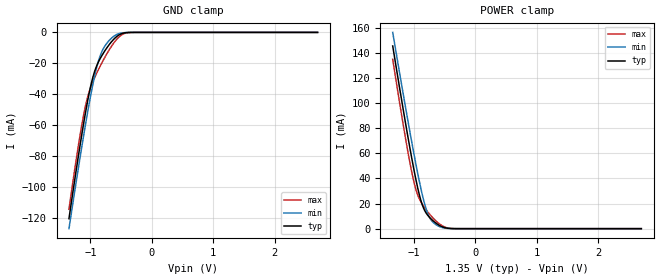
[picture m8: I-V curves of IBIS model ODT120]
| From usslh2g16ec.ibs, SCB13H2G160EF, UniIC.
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|   Model ODT120
[Model]  ODT120
Model_type Input
Vinl =   0.5750V
Vinh =   0.7750V
| variable   typ   min   max
C_comp   1.0500pF   1.0000pF   1.1000pF
| variable   typ   min   max
[Temperature Range]   45.000   95.000   0.000
| variable   typ   min   max
[Voltage Range]   1.35V   1.283V   1.4250V
| variable   typ   min   max
[POWER Clamp Reference] 1.35V   1.283V   1.4250V
| variable   typ   min   max
[GND Clamp Reference]   0.000V   0.000V   0.000V
[Add Submodel]
| Submodel Name   Mode
120ohm_ODT   Non-Driving
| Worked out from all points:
|   GND clamp passes 1 mA (typ) near -0.50 V on its own axis
|   POWER clamp passes 1 mA (typ) near -0.51 V on its own axis
[GND_clamp]
|Voltage   I(typ)   I(min)   I(max)
-1.35V    -120.2mA   -126.6mA   -114.1mA
-1.23V    -88.34mA   -95.9mA    -81.52mA
-1.14V    -65.66mA   -73.61mA   -59.5mA
-1.05V    -45.07mA   -52.44mA   -42.33mA
-990mV    -33.57mA   -39.39mA   -34.75mA
-930mV    -24.92mA   -27.79mA   -29.03mA
-840mV    -16.77mA   -14.89mA   -21.65mA
-750mV    -10.97mA   -7.891mA   -14.99mA
-630mV    -4.83mA    -2.8mA     -7.385mA
-510mV    -1.116mA   -502.7uA   -2.115mA
-360mV    -46.72uA   -22.21uA   -95.74uA
2.7V      0A         0A         0A
[POWER_clamp]
|Voltage   I(typ)   I(min)   I(max)
-1.34V    145.4mA    156.2mA    134.8mA
-1.12V    80.7mA     93.36mA    68.62mA
-1.04V    58.61mA    71.47mA    47.35mA
-980mV    43.17mA    55.66mA    34.17mA
-940mV    33.8mA     45.58mA    27.64mA
-880mV    22.09mA    31.49mA    21.14mA
-800mV    12.67mA    16.11mA    15.22mA
-740mV    8.89mA     8.743mA    11.48mA
-660mV    5.266mA    3.989mA    7.183mA
-520mV    1.208mA    721.2uA    1.904mA
-360mV    46.31uA    30.1uA     72.07uA
2.7V      0A         0A         0A
